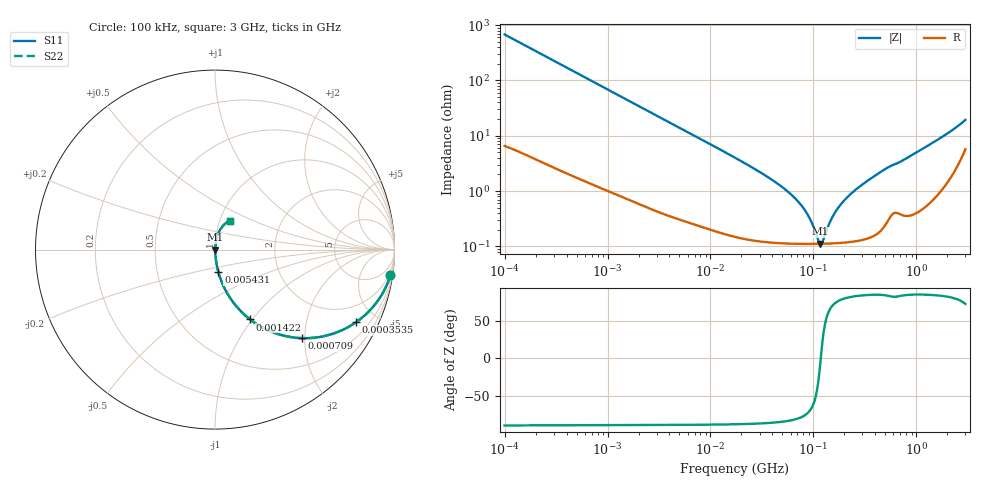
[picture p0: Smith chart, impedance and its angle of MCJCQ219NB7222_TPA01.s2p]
! MCJCQ219NB7222_TPA01  S-PARAMETER MODEL  ( Standard Model )
! Model Generated by TAIYO YUDEN Corporation (http://www.ty-top.com)
! Version 1.0
! TAIYO YUDEN Control No. 220601
! Copyright(c) 2015 TAIYO YUDEN CO.,LTD. All Rights Reserved.
! Product Description (link to TY-COMPAS)
! https://ds.yuden.co.jp/TYCOMPAS/or/detail?pn=MCJCQ219NB7222KTPA01&u=M
! Products Name : Multilayer Ceramic Capacitors
! Characteristics :
!  Capacitance : 2200 [pF] , Rated Voltage : 250 [V] , TCC : X7R
!  Case Size : 2.0 x 1.25 / 0.079 x 0.049 [mm/inch] , Thickness : 0.85 / 0.033 [mm/inch]
!  (Conditions: Temperature = 25 [degC] , DC Bias Voltage = 0 [V])
! External Node Assignments :
!  1  o---| |---o  2
! GND o---------o GND
! Frequency Range : 100kHz  -  3GHz  [ 401 STEP ]
# MHZ S RI R 50
! Freq[MHz].  S11 Real  S11 Imag  S21 Real  S21 Imag  S12 Real  S12 Imag  S22 Real  S22 Imag
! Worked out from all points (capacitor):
!   401 points, 100 kHz to 3 GHz, reference 50 ohm
!   read as one part in series: C = 2.34 nF near 105.3 kHz
!   lowest |Z| = 112 mohm at 116.6 MHz (marker M1)
!   series resonance near 117.9 MHz, so ESL is about 780 pH
!   S11 on the Smith chart (normalised r, x): 100 kHz: 1, -14; 353.5 kHz: 1.05, -3.88; 709 kHz: 1.03, -1.94; 1.422 MHz: 1.02, -0.97; 5.431 MHz: 1.01, -0.26; 3 GHz: 1.11, +0.37
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0.1  0.9774 -0.1437  0.0226 0.1437  0.0226 0.1437  0.9774 -0.1437
0.205778  0.9142 -0.2746  0.0858 0.2746  0.0858 0.2746  0.9142 -0.2746
0.353547  0.787 -0.4035  0.213 0.4035  0.213 0.4035  0.787 -0.4035
0.562235  0.5981 -0.4838  0.4019 0.4838  0.4019 0.4838  0.5981 -0.4838
0.709011  0.4858 -0.4931  0.5142 0.4931  0.5142 0.4931  0.4858 -0.4931
1.421866  0.1957 -0.389  0.8043 0.389  0.8043 0.389  0.1957 -0.389
3.161081  0.05 -0.2088  0.95 0.2088  0.95 0.2088  0.05 -0.2088
5.431059  0.0191 -0.1261  0.9809 0.1261  0.9809 0.1261  0.0191 -0.1261
17.7727  0.00298 -0.0389  0.997 0.0389  0.997 0.0389  0.00298 -0.0389
36.57227  0.00149 -0.0176  0.9985 0.0176  0.9985 0.0176  0.00149 -0.0176
58.15973  0.00121 -0.00926  0.9988 0.00926  0.9988 0.00926  0.00121 -0.00926
79.23846  0.00113 -0.00493  0.9989 0.00493  0.9989 0.00493  0.00113 -0.00493
97.38194  0.00111 -0.00233  0.9989 0.00233  0.9989 0.00233  0.00111 -0.00233
110.7752  0.00111 -0.000756  0.9989 0.000756  0.9989 0.000756  0.00111 -0.000756
116.6348  0.00111 -0.000132  0.9989 0.000132  0.9989 0.000132  0.00111 -0.000132
122.8043  0.00111 0.000491  0.9989 -0.000491  0.9989 -0.000491  0.00111 0.000491
158.9065  0.00115 0.00366  0.9989 -0.00366  0.9989 -0.00366  0.00115 0.00366
200.3904  0.00121 0.00673  0.9988 -0.00673  0.9988 -0.00673  0.00121 0.00673
294.964  0.00146 0.0128  0.9985 -0.0128  0.9985 -0.0128  0.00146 0.0128
547.5153  0.00394 0.0273  0.9961 -0.0273  0.9961 -0.0273  0.00394 0.0273
1791.7  0.0194 0.0926  0.9806 -0.0926  0.9806 -0.0926  0.0194 0.0926
3000  0.0821 0.1606  0.9179 -0.1606  0.9179 -0.1606  0.0821 0.1606
